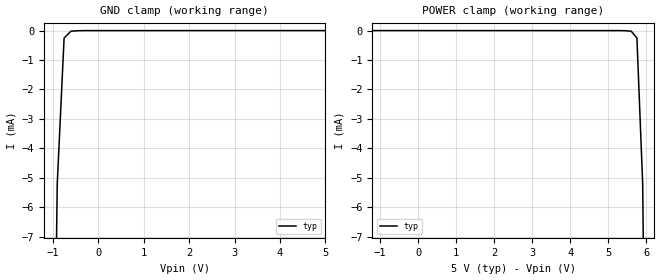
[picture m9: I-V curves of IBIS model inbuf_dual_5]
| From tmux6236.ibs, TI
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| inbuf_dual_5
[Model]   inbuf_dual_5
Model_type   Input
Vinl = 0.8
Vinh = 1.3
|   typ   min   max
C_comp   4.014581e-13   NA   NA
[Voltage Range]   5   NA   NA
[Temperature Range]   27   NA   NA
[Power Clamp Reference]   5   NA   NA
[GND Clamp Reference]   0   NA   NA
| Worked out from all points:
|   GND clamp passes 1 mA (typ) near -0.78 V on its own axis
[GND Clamp]
|   Voltage   I(typ)   I(min)   I(max)
-10V      -2.791A    NA         NA
-1.061V   -23.61mA   NA         NA
-909.1mV  -5.222mA   NA         NA
-757.6mV  -252.3uA   NA         NA
-606.1mV  -20.1uA    NA         NA
5V        683.6nA    NA         NA
[POWER Clamp]
|   Voltage   I(typ)   I(min)   I(max)
-5V       866nA      NA         NA
5.606V    -20.1uA    NA         NA
5.758V    -252.3uA   NA         NA
5.909V    -5.222mA   NA         NA
6.061V    -23.61mA   NA         NA
10V       -1.213A    NA         NA
